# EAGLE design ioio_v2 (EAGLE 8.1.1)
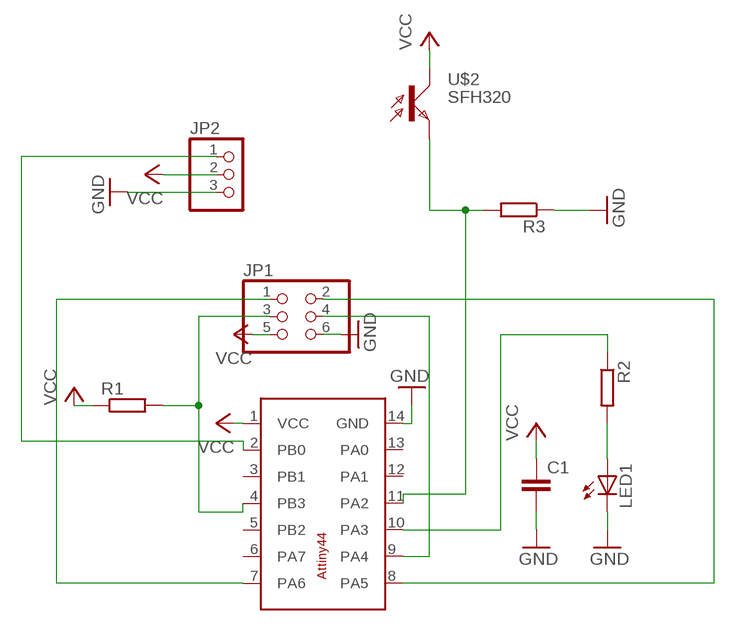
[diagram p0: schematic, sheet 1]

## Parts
C1  C-EUC1206  [C1206]
JP1  PINHD-2X3  [2X03]
JP2  PINHD-1X3  [1X03]
LED1  LEDCHIPLED_1206  [CHIPLED_1206]
R1  R-EU_R1206  [R1206]
R2  R-EU_R1206  [R1206]
R3  R-EU_R1206  [R1206]
U$1  ATTINY44-SO14  [SO14]
U$2  SFH320  [PLCC2]

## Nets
GND: C1.2 JP1.6 JP2.3 LED1.C R3.1 U$1.14(GND)
N$3: JP1.3 R1.2 U$1.4(PB3)
N$4: JP1.1 U$1.7(PA6)
N$5: JP1.2 U$1.8(PA5)
N$6: JP1.4 U$1.9(PA4)
N$7: LED1.A R2.2
N$8: R2.1 U$1.10(PA3)
N$9: R3.2 U$1.11(PA2) U$2.P$1(E)
N$10: JP2.1 U$1.2(PB0)
VCC: C1.1 JP1.5 JP2.2 R1.1 U$1.1(VCC) U$2.P$2(C)
Unconnected: U$1.3(PB1) U$1.5(PB2) U$1.6(PA7) U$1.12(PA1) U$1.13(PA0)

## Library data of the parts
C1 = rcl:C-EU: CAPACITOR, European symbol
JP1 = pinhead:PINHD-2X3: PIN HEADER
JP2 = pinhead:PINHD-1X3: PIN HEADER
LED1 = led:LED: LED
R1-R3 = resistor:R-EU_: RESISTOR, European symbol
U$1 = atmel-new:ATTINY44-SO14
U$2 = PLCC2:SFH320

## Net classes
0 default: width 0.61 mm

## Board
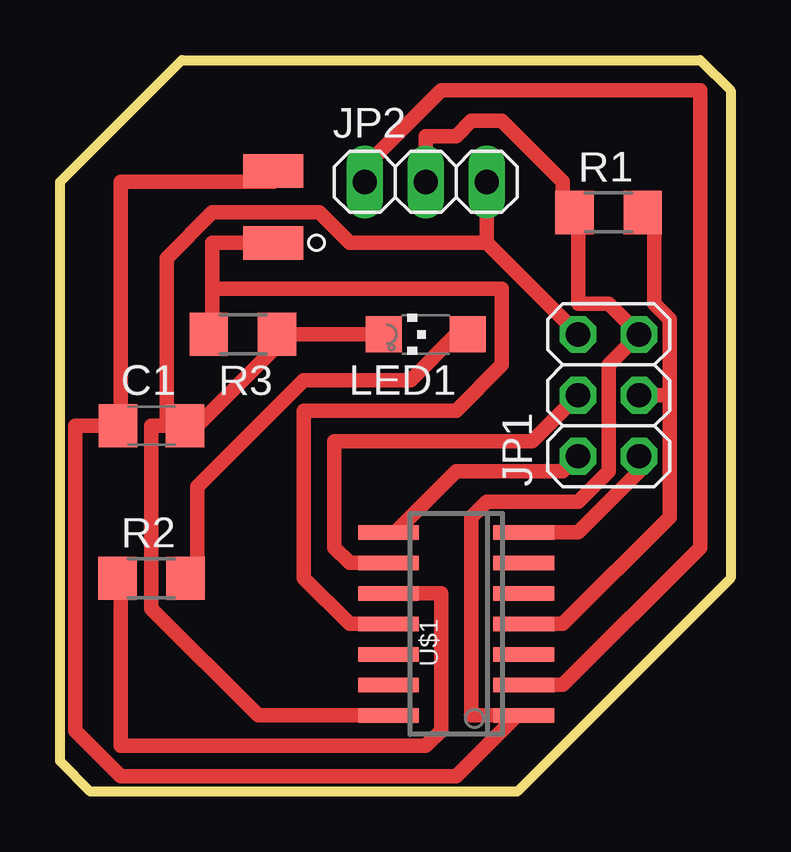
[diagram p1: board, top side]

Size 27.94 x 30.48 mm. Coordinates in mm from the lower left corner, seen from the top.
Outline: 0,25.4 5.08,30.48 26.67,30.48 27.94,29.21 27.94,8.89 19.05,0 1.27,0 0,1.27 0,25.4
Copper layers (1*16): Top 0.035mm / dielectric 1.5mm / Bottom 0.035mm
Design rules "default": minimum track width 10mil, minimum drill 24mil, track to track 8mil, track to pad 8mil, pad to pad 8mil, via to via 8mil, smd to smd 8mil, copper to edge 40mil, drill to drill 8mil, minimum pad ring 10mil, minimum via ring 8mil, stop-mask expansion 4mil, vias tented up to drill 0mil, thermal gap 10mil

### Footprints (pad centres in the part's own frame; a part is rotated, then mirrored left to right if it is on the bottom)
C1206 = smd 1.6 x 1.8: 1 -1.4,0; 2 1.4,0
2X03 = drill 1.016 octagon: 1 -2.54,-1.27; 2 -2.54,1.27; 3 0,-1.27; 4 0,1.27; 5 2.54,-1.27; 6 2.54,1.27
1X03 = drill 1.016 long: 1 -2.54,0; 2 0,0; 3 2.54,0
CHIPLED_1206 = smd 1.5 x 1.5: A 0,-1.75; C 0,1.75
R1206 = smd 1.6 x 1.803: 1 -1.422,0; 2 1.422,0
SO14 = smd 0.6 x 2.54: 1 -3.175,-2.822; 2 -1.905,-2.822; 3 -0.635,-2.822; 4 0.635,-2.822; 5 1.905,-2.822; 6 3.175,-2.822; 7 4.445,-2.822; 8 4.445,2.822; 9 3.175,2.822; 10 1.905,2.822; 11 0.635,2.822; 12 -0.635,2.822; 13 -1.905,2.822; 14 -3.175,2.822
PLCC2 = smd 2.5 x 1.4: P$1 0,0; P$2 0,-3

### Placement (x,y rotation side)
C1  3.81,15.24 0 top
JP1  22.86,16.51 90 top
JP2  15.24,25.4 0 top
LED1  15.24,19.05 90 top
R1  22.86,24.13 0 top
R2  3.81,8.89 0 top
R3  7.62,19.05 180 top
U$1  16.51,6.35 90 top
U$2  8.89,22.86 180 top

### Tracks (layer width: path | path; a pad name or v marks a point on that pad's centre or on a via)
GND
  Top 0.61: 17.78,22.86 JP1.6 | JP2.3 17.78,22.86 | 9.53,19.05 LED1.C | 9.53,19.05 5.72,15.24 C1.2 | 9.53,19.05 R3.1 | U$1.14 8.26,3.17 3.81,7.62 3.81,15.24 4.45,15.24 | C1.2 4.45,15.24 | 17.78,22.86 12.06,22.86 10.8,24.13 6.35,24.13 4.45,22.23 4.45,15.24 | 5.08,15.24 C1.2
N$3
  Top 0.61: 25.4,16.51 25.4,19.68 24.77,20.32 24.77,24.13 R1.2 | JP1.3 25.4,16.51 | U$1.4 20.95,6.98 25.4,11.43 25.4,16.51
N$4
  Top 0.61: U$1.7 21.59,10.8 24.13,13.34 JP1.1
N$5
  Top 0.61: JP1.2 20.95,13.34 16.51,13.34 13.97,10.8 U$1.8
N$6
  Top 0.61: U$1.9 12.06,9.52 11.43,10.16 11.43,14.6 19.69,14.6 JP1.4
N$7
  Top 0.61: LED1.A 16.51,19.05 14.61,17.14 10.16,17.14 5.72,12.7 5.72,8.89 R2.2
N$8
  Top 0.61: U$1.10 15.88,8.25 15.88,2.54 15.24,1.91 2.54,1.91 2.54,8.89 R2.1
N$9
  Top 0.61: 6.35,20.95 6.35,22.86 U$2.P$1 | 6.35,20.95 6.35,19.05 R3.2 | U$1.11 12.06,6.98 10.16,8.89 10.16,15.88 16.51,15.88 18.42,17.78 18.42,20.95 6.35,20.95
N$10
  Top 0.61: U$1.2 20.95,4.45 26.67,10.16 26.67,29.21 15.88,29.21 12.7,26.04 JP2.1
VCC
  Top 0.61: JP2.2 15.24,27.3 16.51,27.3 17.15,27.94 18.42,27.94 20.95,25.4 20.95,24.13 R1.1 21.59,24.13 21.59,20.32 22.86,20.32 JP1.5 22.86,17.78 22.86,13.34 21.59,12.06 17.78,12.06 17.15,11.43 17.15,3.17 19.05,3.17 | U$2.P$2 8.89,25.4 2.54,25.4 2.54,15.24 C1.1 0.64,15.24 0.64,2.54 2.54,0.63 16.51,0.63 19.05,3.17 | 19.05,3.17 U$1.1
